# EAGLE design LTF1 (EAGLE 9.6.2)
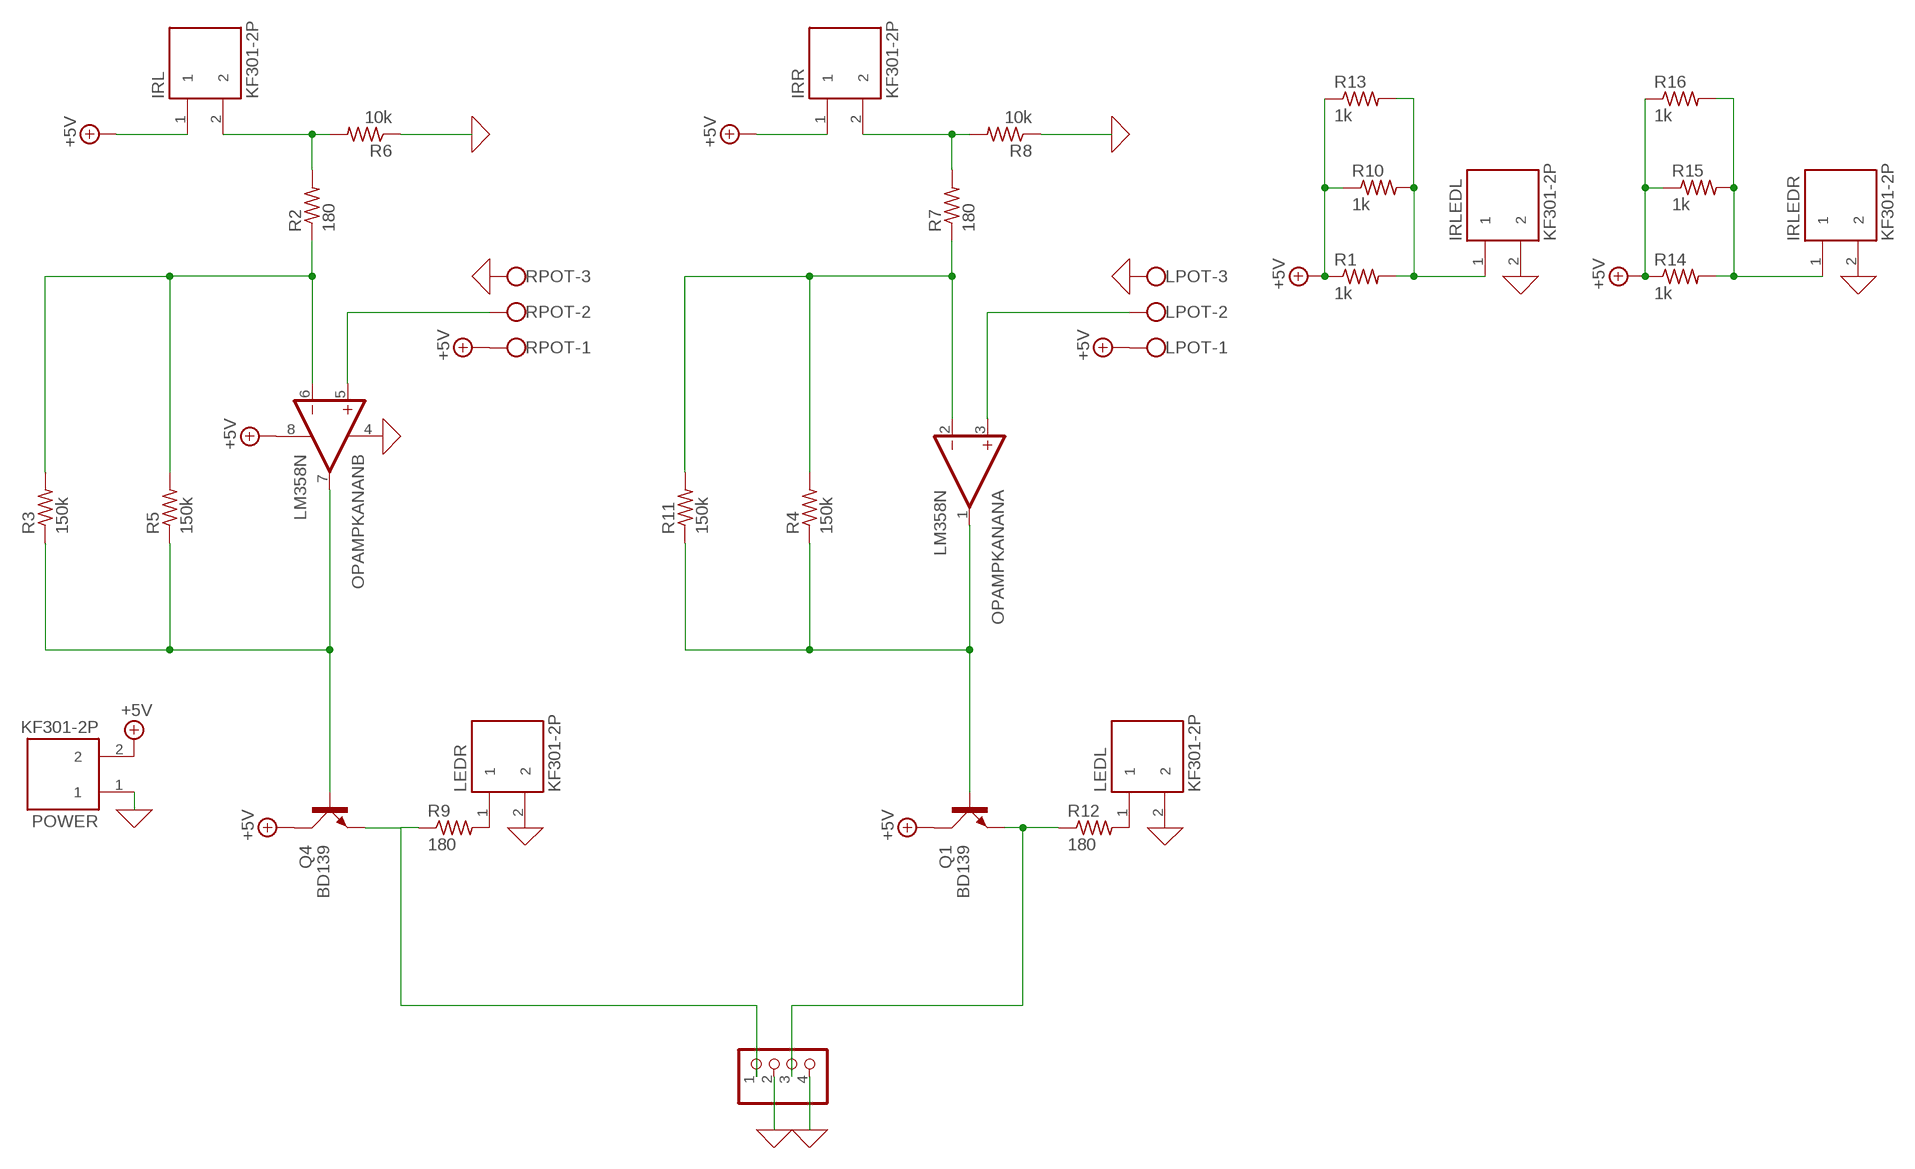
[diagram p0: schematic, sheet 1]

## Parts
IRL  KF301-2P  [HANDSON_KF301-2P]
IRLEDL  KF301-2P  [HANDSON_KF301-2P]
IRLEDR  KF301-2P  [HANDSON_KF301-2P]
IRR  KF301-2P  [HANDSON_KF301-2P]
LEDL  KF301-2P  [HANDSON_KF301-2P]
LEDR  KF301-2P  [HANDSON_KF301-2P]
LPOT  W237-103  [W237-103]
MOTORDRIVER  PINHD-1X4  [1X04]
OPAMPKANAN  LM358N  [DIL08]
POWER  KF301-2P  [HANDSON_KF301-2P]
Q1  BD139  [TO126AV]
Q4  BD139  [TO126AV]
R1  1k  R-US_0204/7  [0204/7]
R2  180  R-US_0204/7  [0204/7]
R3  150k  R-US_0204/7  [0204/7]
R4  150k  R-US_0204/7  [0204/7]
R5  150k  R-US_0204/7  [0204/7]
R6  10k  R-US_0204/7  [0204/7]
R7  180  R-US_0204/7  [0204/7]
R8  10k  R-US_0204/7  [0204/7]
R9  180  R-US_0204/7  [0204/7]
R10  1k  R-US_0204/7  [0204/7]
R11  150k  R-US_0204/7  [0204/7]
R12  180  R-US_0204/7  [0204/7]
R13  1k  R-US_0204/7  [0204/7]
R14  1k  R-US_0204/7  [0204/7]
R15  1k  R-US_0204/7  [0204/7]
R16  1k  R-US_0204/7  [0204/7]
RPOT  W237-103  [W237-103]

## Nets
0: IRLEDL.2 IRLEDR.2 LEDL.2 LEDR.2 LPOT.3 MOTORDRIVER.2 MOTORDRIVER.4 OPAMPKANAN.4(P:V-) POWER.1 R6.1 R8.1 RPOT.3 ; supply symbol labelled GND
+5V: IRL.1 IRR.1 LPOT.1 OPAMPKANAN.8(P:V+) POWER.2 Q1.C Q4.C R1.1 R10.1 R13.1 R14.1 R15.1 R16.1 RPOT.1
IRKIRI: IRL.2 R2.2 R6.2
LEDIRKANAN: IRLEDL.1 R1.2 R10.2 R13.2
LEDIRKANAN1: IRLEDR.1 R14.2 R15.2 R16.2
MOTORKANAN: OPAMPKANAN.7(B:OUT) Q4.B R3.1 R5.1
MOTORKANAN1: OPAMPKANAN.1(A:OUT) Q1.B R4.1 R11.1
N$1: LEDR.1 R9.2
N$2: LEDL.1 R12.2
N$3: OPAMPKANAN.2(A:-IN) R4.2 R7.1 R11.2
N$4: LPOT.2 OPAMPKANAN.3(A:+IN)
N$5: IRR.2 R7.2 R8.2
N$6: MOTORDRIVER.3 Q1.E R12.1
N$7: OPAMPKANAN.6(B:-IN) R2.1 R3.2 R5.2
N$8: MOTORDRIVER.1 Q4.E R9.1
N$10: OPAMPKANAN.5(B:+IN) RPOT.2

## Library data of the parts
IRL IRLEDL IRLEDR IRR LEDL LEDR POWER = KF301-2P:KF301-2P: 2 Pin Terminal Block 5mm Pitch Check availability; AVAILABILITY: Not in stock; DESCRIPTION: 2 Pin Terminal Block 5mm Pitch; MF: Handson Technology; MP: KF301-2P; PACKAGE: None; PRICE: None
LPOT RPOT = con-wago-500:W237-103: WAGO SCREW CLAMP; MPN: 237-103; OC_FARNELL: unknown; OC_NEWARK: 18M7116
MOTORDRIVER = pinhead:PINHD-1X4: PIN HEADER
OPAMPKANAN = linear:LM358: OP AMP also LM158; LM258; LM2904 Source: http://cache.national.com/ds/LM/LM158.pdf
Q1 Q4 = transistor-power:BD139: NPN TRANSISTOR
R1-R16 = rcl:R-US_: RESISTOR, American symbol; SPICEPREFIX: R

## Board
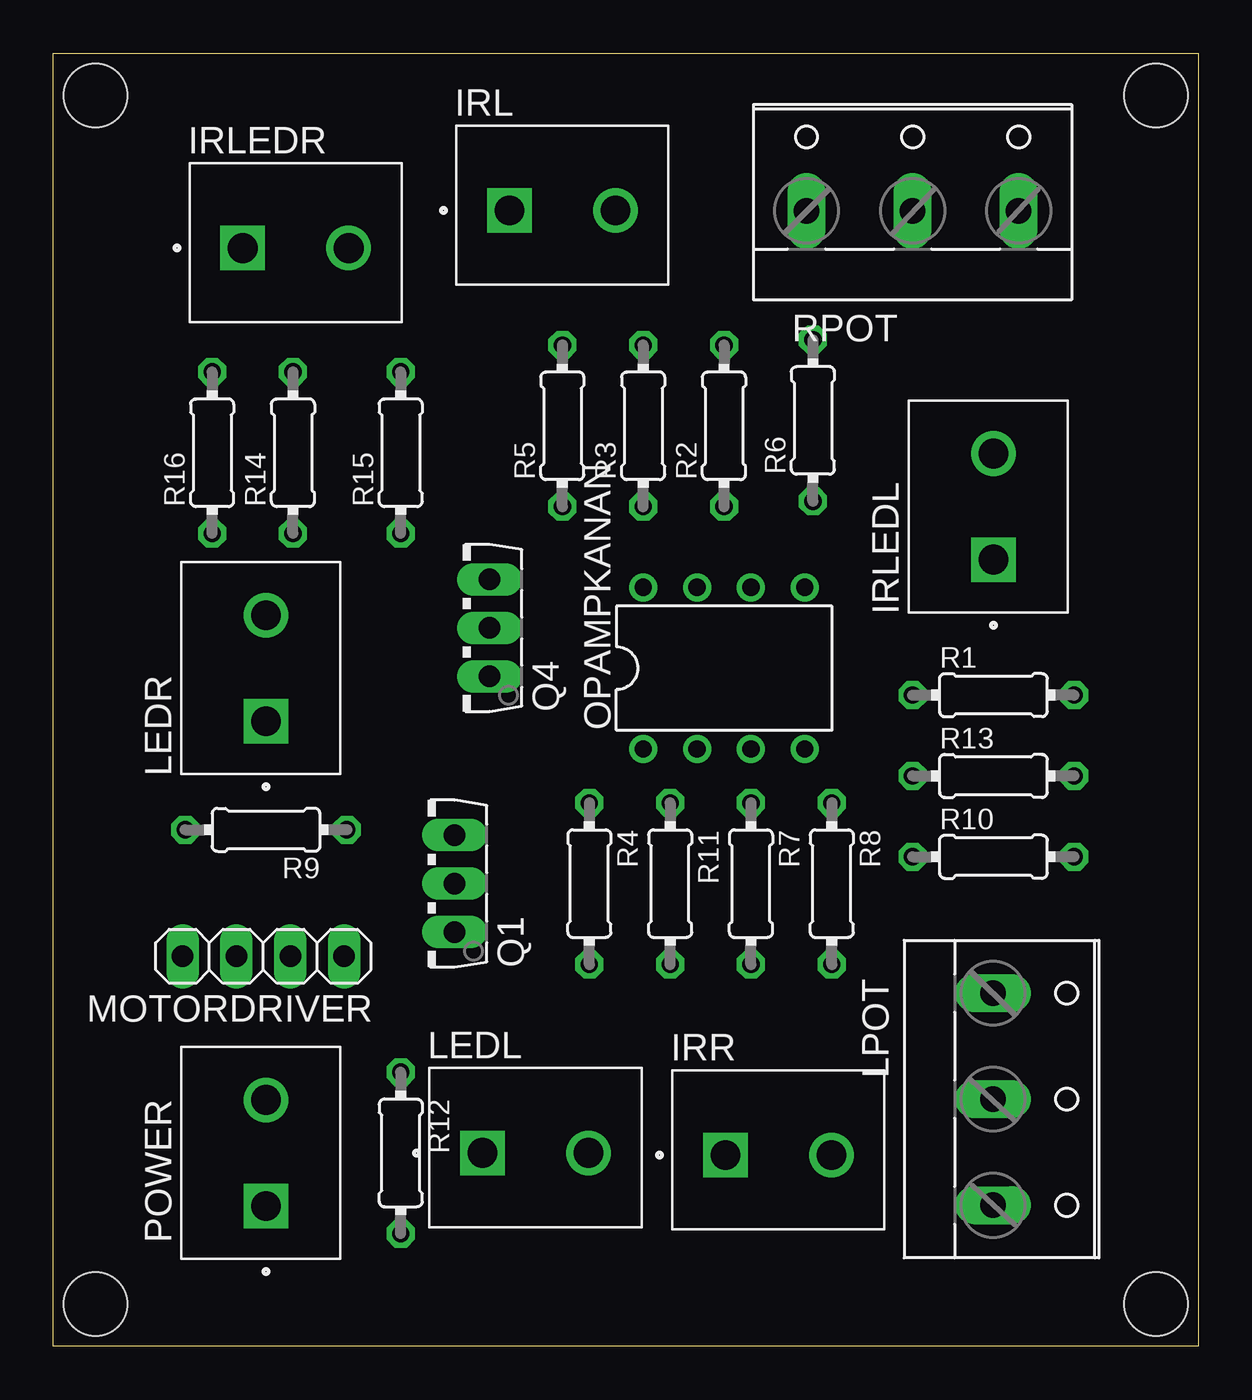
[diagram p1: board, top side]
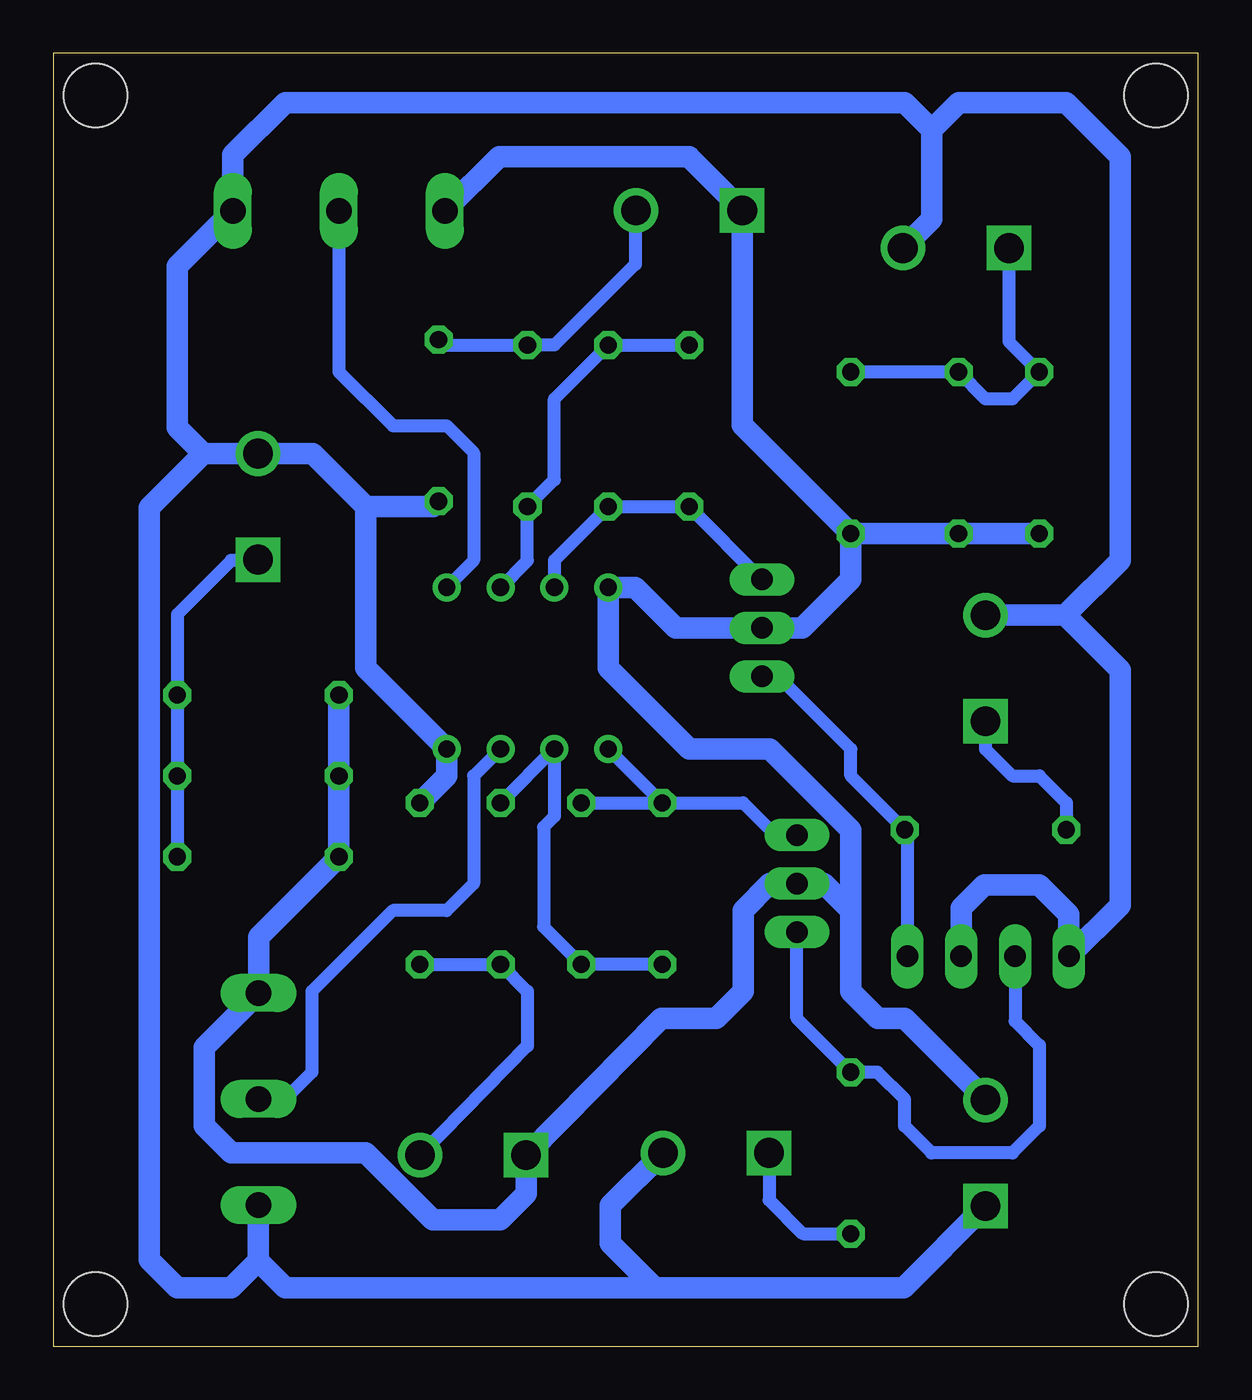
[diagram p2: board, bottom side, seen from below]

Size 54 x 61 mm. Coordinates in mm from the lower left corner, seen from the top.
Outline: 0,0 0,61 54,61 54,0 0,0
Copper layers (1*16): Top 0.035mm / dielectric 1.5mm / Bottom 0.035mm
Design rules "default": minimum track width 6mil, minimum drill 0.35mm, track to track 6mil, track to pad 6mil, pad to pad 6mil, via to via 6mil, smd to smd 6mil, copper to edge 40mil, drill to drill 6mil, minimum pad ring 10mil, minimum via ring 8mil, stop-mask expansion 4mil, vias tented up to drill 0mil, thermal gap 10mil
Holes 3 mm at 2,2 52,2 52,59 2,59

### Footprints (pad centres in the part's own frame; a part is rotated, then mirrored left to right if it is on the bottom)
HANDSON_KF301-2P = drill 1.4 square: 1 -2.5,0 | drill 1.4: 2 2.5,0
W237-103 = drill 1.194 long: 1 -5,-1.29; 2 0,-1.29; 3 5,-1.29
1X04 = drill 1.016 long: 1 -3.81,0; 2 -1.27,0; 3 1.27,0; 4 3.81,0
DIL08 = drill 0.813 pad 1.27: 1 -3.81,-3.81; 2 -1.27,-3.81; 3 1.27,-3.81; 4 3.81,-3.81; 5 3.81,3.81; 6 1.27,3.81; 7 -1.27,3.81; 8 -3.81,3.81
TO126AV = drill 1.016 long: B 2.286,-1.27; C 0,-1.27; E -2.286,-1.27
0204/7 = drill 0.813 octagon: 1 -3.81,0; 2 3.81,0

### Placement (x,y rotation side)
IRL  24.01,53.58 0 top
IRLEDL  44.33,39.61 90 top
IRLEDR  11.44,51.8 0 top
IRR  34.2,9.03 0 top
LEDL  22.74,9.13 0 top
LEDR  10.04,31.99 90 top
LPOT  45.6,11.67 270 top
MOTORDRIVER  9.92,18.4 180 top
OPAMPKANAN  31.63,31.99 0 top
POWER  10.04,9.13 90 top
Q1  17.66,21.83 90 top
Q4  19.31,33.89 90 top
R1  44.33,30.72 0 top
R2  31.63,43.42 90 top
R3  27.82,43.42 90 top
R4  25.28,21.83 270 top
R5  24.01,43.42 90 top
R6  35.82,43.67 90 top
R7  32.9,21.83 270 top
R8  36.71,21.83 270 top
R9  10.04,24.37 180 top
R10  44.33,23.1 0 top
R11  29.09,21.83 270 top
R12  16.39,9.13 270 top
R13  44.33,26.91 0 top
R14  11.31,42.15 90 top
R15  16.39,42.15 90 top
R16  7.5,42.15 90 top
RPOT  40.52,54.85 0 top

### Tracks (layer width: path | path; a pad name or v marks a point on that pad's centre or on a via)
0
  Bottom 1.016: POWER.1 13.89,2.78 25.64,2.78 | 44.33,4.05 43.06,2.78 25.64,2.78 | 44.33,4.05 44.33,6.65 LPOT.3 | 44.33,4.05 45.6,2.78 48.14,2.78 49.46,4.1 49.46,39.56 46.91,42.11 | 46.91,42.11 IRLEDL.2 41.75,42.11 39.25,39.61 | 39.25,39.61 36.08,39.61 R6.1 | 39.25,39.61 39.25,31.99 OPAMPKANAN.4 35.44,26.91 R8.1 | 46.91,42.11 48.14,43.34 48.14,50.94 RPOT.3 45.52,56.2 43.06,58.66 13.85,58.66 12.58,57.39 | 12.58,57.39 12.58,53.16 IRLEDR.2 | 12.58,57.39 11.31,58.66 6.23,58.66 3.69,56.12 3.69,37.07 6.27,34.49 | LEDR.2 6.27,34.49 | 6.27,34.49 3.69,31.91 3.69,20.81 MOTORDRIVER.4 6.11,20.38 7.5,21.78 10.09,21.78 11.19,20.68 MOTORDRIVER.2 | LEDL.2 27.72,6.65 27.72,4.86 25.64,2.78
+5V
  Bottom 1.016: POWER.2 10.04,11.67 13.85,15.48 15.12,15.48 16.39,16.75 16.39,20.56 | 16.39,20.56 17.66,21.83 Q1.C 20.2,21.83 21.47,20.56 21.47,16.75 22.74,15.48 25.32,15.48 IRR.1 31.7,7.21 32.93,5.98 36.1,5.98 39.25,9.13 45.6,9.13 46.87,10.4 46.87,14.11 LPOT.1 44.31,19.31 R10.1 R13.1 R1.1 | RPOT.1 32.96,56.12 24.01,56.12 24.01,56.08 IRL.1 21.51,43.46 R15.1 | R15.1 R14.1 R16.1 | 16.39,20.56 16.39,24.37 20.2,28.18 24.01,28.18 27.82,31.99 OPAMPKANAN.8 26.55,35.8 24.65,33.89 Q4.C 18.68,33.89 16.39,36.18 R15.1
IRKIRI
  Bottom 0.61: R6.2 35.57,47.23 R2.2 30.36,47.23 26.55,51.04 26.55,53.54 IRL.2
LEDIRKANAN
  Bottom 0.61: IRLEDL.1 44.37,37.07 45.6,37.07 48.14,34.53 R1.2 R13.2 R10.2
LEDIRKANAN1
  Bottom 0.61: IRLEDR.1 8.94,47.4 R16.2 8.77,44.69 10.04,44.69 R14.2 R15.2
MOTORKANAN
  Bottom 0.61: OPAMPKANAN.7 30.36,37.07 R3.1 R5.1 Q4.B
MOTORKANAN1
  Bottom 0.61: Q1.B 19.95,24.11 21.47,25.64 R4.1 | OPAMPKANAN.1 R4.1 | R11.1 R4.1
N$1
  Bottom 0.61: LEDR.1 10.04,28.18 8.77,26.91 7.5,26.91 6.23,25.64 R9.2
N$2
  Bottom 0.61: LEDL.1 20.24,6.91 18.65,5.32 R12.2
N$3
  Bottom 0.61: R4.2 R11.2 30.87,19.8 30.87,24.5 30.36,25 OPAMPKANAN.2 R7.1
N$4
  Bottom 0.61: OPAMPKANAN.3 34.17,26.91 34.17,21.83 35.44,20.56 37.98,20.56 41.79,16.75 41.79,12.94 43.06,11.67 LPOT.2
N$5
  Bottom 0.61: R8.2 R7.2 31.63,16.75 31.63,14.17 IRR.2
N$6
  Bottom 0.61: Q1.E 18.93,15.48 R12.1 15.12,12.94 13.85,11.67 13.85,10.4 12.58,9.13 8.77,9.13 7.5,10.4 7.5,14.21 8.64,15.35 MOTORDRIVER.3
N$7
  Bottom 0.61: OPAMPKANAN.6 31.63,37.07 R2.1 30.36,40.88 30.36,44.69 R3.2 R5.2
N$8
  Bottom 0.61: MOTORDRIVER.1 13.72,24.24 R9.1 16.39,26.91 16.39,28.18 19.82,31.61 Q4.E
N$10
  Bottom 0.61: RPOT.2 40.52,45.96 37.98,43.42 35.44,43.42 34.17,42.15 34.17,37.07 OPAMPKANAN.5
